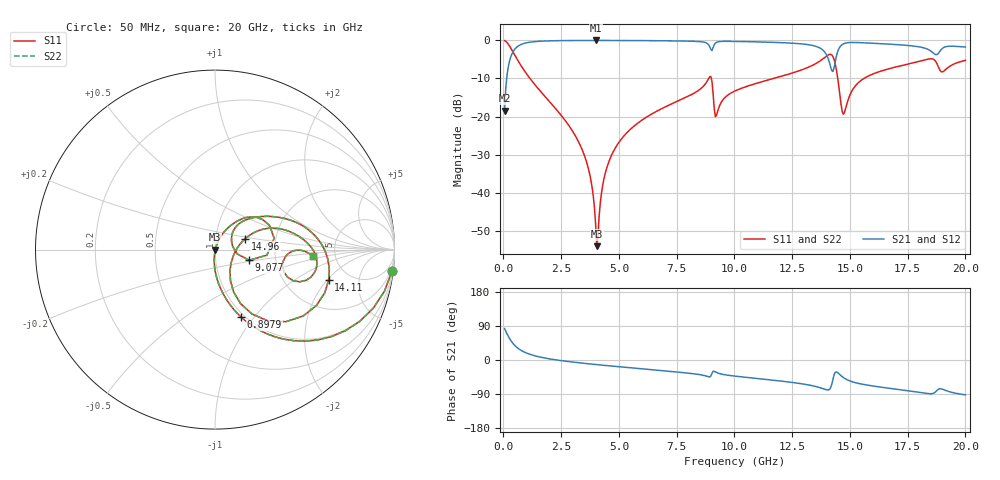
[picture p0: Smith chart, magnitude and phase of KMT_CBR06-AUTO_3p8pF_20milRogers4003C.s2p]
! Data measured by Modelithics Inc. support@modelithics.com 813-866-6335
! KEMET CBR06-AUTO 3.8pF, Pad Width= 0.851mm, Pad Length= 0.64mm, Pad Gap= 0.62mm, 20mil Rogers 4003C substrate Data, January 2022
# hz S ma R 50
! 2 Port Network Data from SP1.SP block
! freq  magS11  angS11  magS21  angS21  magS12  angS12  magS22  angS22
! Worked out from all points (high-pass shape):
!   401 points, 50 MHz to 20 GHz, reference 50 ohm
!   highest |S21| = -0.02 dB at 3.99 GHz (marker M1); lowest = -18.5 dB at 50 MHz (marker M2)
!   |S21| within 3 dB of the highest: 412.6 MHz to 13.9 GHz (13.49 GHz wide, 188 % of centre); 14.47 GHz to 18.55 GHz (4.085 GHz wide, 24.7 % of centre)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
!   lowest |S11| = -54.0 dB at 4.04 GHz (marker M3), VSWR 1.00, Z = 50.2 - j0.116 ohm
!   |S11| at or under -10 dB: 1.149 GHz to 8.885 GHz (7.736 GHz wide, 154 % of centre); 8.998 GHz to 11.69 GHz (2.689 GHz wide, 26 % of centre); 14.47 GHz to 15.61 GHz (1.133 GHz wide, 7.53 % of centre)
!   |S22| runs from -54.0 to -0.1 dB; largest |S21 - S12| = 0
!   S11 on the Smith chart (normalised r, x): 50 MHz: 1, -16; 897.9 MHz: 0.96, -0.86; 9.077 GHz: 1.46, -0.18; 14.11 GHz: 3.49, -2.08; 14.96 GHz: 1.39, +0.18; 20 GHz: 3.37, -0.36
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5e7  0.9928 -7.0  0.1194 83.0  0.1194 83.0  0.9928 -7.0
3.4925e8  0.7629 -41.3  0.6456 48.7  0.6456 48.7  0.7629 -41.3
8.97875e8  0.4032 -68.8  0.9141 21.1  0.9141 21.1  0.4032 -68.8
3.391625e9  0.0378 -95.5  0.9975 -8.1  0.9975 -8.1  0.0378 -95.5
3.74075e9  0.01718 -94.4  0.998 -10.3  0.998 -10.3  0.01718 -94.4
3.990125e9  0.00388 -73.9  0.998 -11.9  0.998 -11.9  0.00388 -73.9
4.04e9  0.001994 -35.3  0.998 -12.2  0.998 -12.2  0.001994 -35.3
4.389125e9  0.01712 69.3  0.9978 -14.2  0.9978 -14.2  0.01712 69.3
4.788125e9  0.0362 70.3  0.9972 -16.5  0.9972 -16.5  0.0362 70.3
6.73325e9  0.1219 61.5  0.9897 -27.3  0.9897 -27.3  0.1219 61.5
8.877875e9  0.3136 32.2  0.8795 -44.4  0.8795 -44.4  0.3136 32.2
9.077375e9  0.1995 -17.3  0.8039 -29.7  0.8039 -29.7  0.1995 -17.3
9.227e9  0.1045 28.7  0.9459 -33.0  0.9459 -33.0  0.1045 28.7
1.0025e10  0.217 45.8  0.9697 -42.6  0.9697 -42.6  0.217 45.8
1.336662e10  0.4684 19.5  0.8603 -67.7  0.8603 -67.7  0.4684 19.5
1.411475e10  0.6555 -15.0  0.5109 -77.6  0.5109 -77.6  0.6555 -15.0
1.436412e10  0.4933 -53.5  0.5232 -32.5  0.5232 -32.5  0.4933 -53.5
1.471325e10  0.1075 -22.2  0.9003 -46.2  0.9003 -46.2  0.1075 -22.2
1.496262e10  0.1794 19.9  0.9359 -54.4  0.9359 -54.4  0.1794 19.9
1.670825e10  0.4257 13.8  0.8927 -74.7  0.8927 -74.7  0.4257 13.8
1.875312e10  0.5054 -20.8  0.6495 -81.5  0.6495 -81.5  0.5054 -20.8
2e10  0.5466 -3.9  0.8184 -92.0  0.8184 -92.0  0.5466 -3.9
